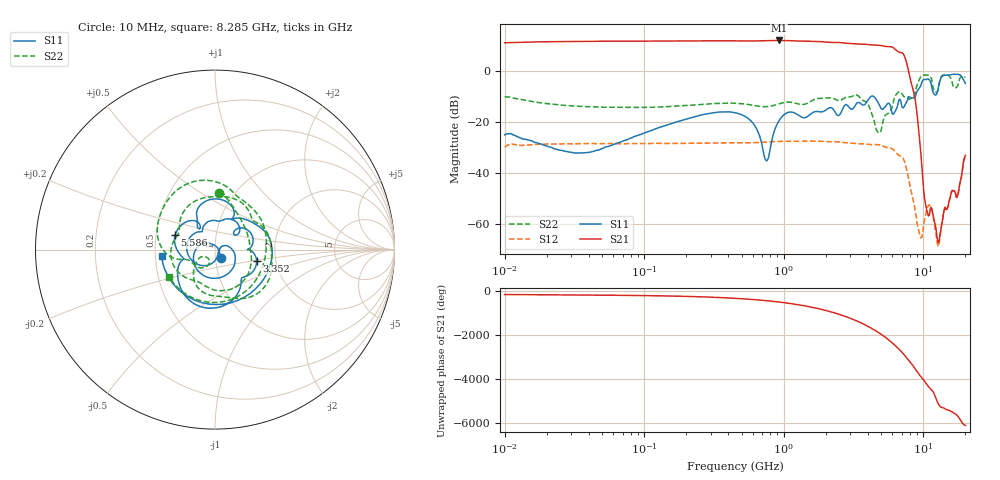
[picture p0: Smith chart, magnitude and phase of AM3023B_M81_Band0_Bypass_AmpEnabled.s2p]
!Agilent Technologies,E8364B,MY43040894,A.07.50.67
!Agilent E8364B: A.07.50.67
!Date: Tuesday, October 27, 2020 10:41:50
!Correction: S11(Full 2 Port(1,2))
!S21(Full 2 Port(1,2))
!S12(Full 2 Port(1,2))
!S22(Full 2 Port(1,2))
!S2P File: Measurements: S11, S21, S12, S22:Log Frequency Sweep
# Hz S  dB  R 50
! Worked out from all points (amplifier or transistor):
!   3201 points, 10 MHz to 20 GHz, reference 50 ohm
!   highest |S21| = 12.2 dB at 925.1 MHz (marker M1)
!   |S21| within 3 dB of that: start of sweep to 6.139 GHz
!   unconditionally stable (mu >= 1): start of sweep to end of sweep
!   at 35.47 MHz: K = 3.30, MAG = 12.0 dB, |S12| = -28.4 dB
!   at 447.2 MHz: K = 2.99, MAG = 12.4 dB, |S12| = -28.1 dB
!   at 20 GHz: K = 287.17, MAG = -27.4 dB, |S12| = -33.5 dB
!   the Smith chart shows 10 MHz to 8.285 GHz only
!   S11 on the Smith chart (normalised r, x): 10 MHz: 1.06, -0.10; 3.352 GHz: 1.59, -0.22; 5.586 GHz: 0.63, +0.11; 8.285 GHz: 0.54, -0.04
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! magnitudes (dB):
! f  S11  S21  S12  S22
! 10 MHz  -24.9  11.3  -29.8  -10.0
! 35.55 MHz  -32.0  11.8  -28.4  -13.8
! 126.1 MHz  -22.2  11.9  -28.3  -14.0
! 447.2 MHz  -16.2  12.0  -28.1  -12.5
! 613.4 MHz  -21.0  12.0  -28.0  -13.4
! 750.6 MHz  -35.1  12.1  -27.8  -13.9
! 925.1 MHz  -19.4  12.2  -27.5  -12.8
! 1.59 GHz  -16.4  11.8  -27.5  -11.5
! 3.352 GHz  -12.4  10.8  -28.4  -9.3
! 4.764 GHz  -12.5  10.3  -28.8  -24.0
! 5.586 GHz  -12.5  9.8  -30.1  -16.5
! 5.639 GHz  -12.5  9.8  -30.1  -16.4
! 7.202 GHz  -14.2  6.8  -34.5  -9.8
! 8.285 GHz  -10.4  -5.7  -48.7  -10.5
! 9.509 GHz  -6.0  -30.0  -65.2  -2.4
! 10.41 GHz  -3.2  -52.7  -56.3  -1.4
! 11.28 GHz  -4.3  -53.8  -53.3  -2.3
! 12.74 GHz  -7.2  -67.4  -68.6  -7.3
! 13.87 GHz  -1.7  -56.5  -56.5  -1.4
! 15.85 GHz  -1.3  -47.6  -47.7  -3.2
! 17.76 GHz  -1.2  -48.1  -48.1  -5.1
! 20 GHz  -4.7  -33.0  -33.5  -2.3
